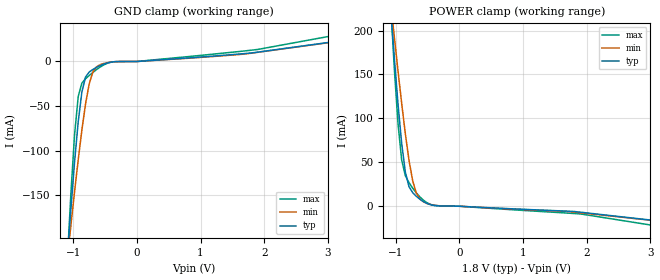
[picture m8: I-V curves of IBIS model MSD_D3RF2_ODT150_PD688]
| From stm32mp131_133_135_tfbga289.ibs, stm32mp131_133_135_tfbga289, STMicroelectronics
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[Model] MSD_D3RF2_ODT150_PD688
Model_type   Input
C_comp 2.387pF   2.319pF   2.454pF
Vinh = 1.150V
Vinl = 650.000mV
[Temperature Range]   25.000   125.000   -40.000
[Voltage Range]   1.800V   1.700V   1.900V
[GND Clamp Reference]   0.00V   0.00V   0.00V
[POWER Clamp Reference]   1.800V   1.700V   1.900V
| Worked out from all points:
|   GND clamp passes 1 mA (typ) near -0.43 V on its own axis
|   POWER clamp passes 1 mA (typ) near -0.40 V on its own axis
[GND Clamp]
-1.785V   -949.2mA   -706.9mA   -1.312A
-1.094V   -221.3mA   -222.3mA   -226mA
-1.036V   -165.3mA   -183.8mA   -148mA
-978.8mV  -113.1mA   -146.3mA   -82.53mA
-921.2mV  -67.68mA   -110.4mA   -39.29mA
-863.6mV  -34.21mA   -76.88mA   -24.21mA
-806.1mV  -17.43mA   -47.59mA   -19.39mA
-748.5mV  -11.81mA   -25.06mA   -15.69mA
-690.9mV  -8.945mA   -11.69mA   -12.25mA
-575.8mV  -4.581mA   -3.565mA   -6.192mA
1.9V      10.53mA    10.33mA    13.54mA
3.57V     26.85mA    26.52mA    35.41mA
[Power Clamp]
-1.77V    960.5mA    723.6mA    1.316A
-1.079V   225mA      231.8mA    230.2mA
-1.021V   168.6mA    192.6mA    156.2mA
-963.6mV  116.3mA    154.2mA    94.17mA
-906.1mV  71.57mA    117.1mA    52.55mA
-848.5mV  38.86mA    82.51mA    34.72mA
-790.9mV  22.23mA    52.23mA    26.81mA
-733.3mV  15.51mA    29.02mA    20.61mA
-675.8mV  11.31mA    14.92mA    15.17mA
-560.6mV  5.111mA    4.871mA    6.662mA
1.915V    -6.917mA   -7.588mA   -8.916mA
3.585V    -20.48mA   -20.49mA   -28.07mA
